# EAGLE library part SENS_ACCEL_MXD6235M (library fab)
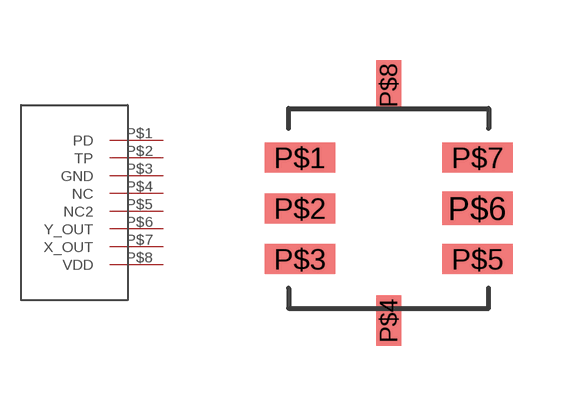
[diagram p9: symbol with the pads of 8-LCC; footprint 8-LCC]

Designator prefix -

## SENS_ACCEL_MXD6235M-SMD  [8-LCC]
P$1  PD
P$2  TP
P$3  GND  pwr
P$4  NC  nc
P$5  NC2  nc
P$6  Y_OUT
P$7  X_OUT
P$8  VDD  pwr

## Footprint 8-LCC (pad centres in mm)
smd 1.77 x 0.75: P$1 -2.22,1.27; P$2 -2.22,0; P$3 -2.22,-1.27; P$5 2.22,-1.27; P$7 2.22,1.27
smd 0.635 x 1.27: P$4 0,-2.81; P$8 0,3.08
smd 1.77 x 0.84: P$6 2.22,0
